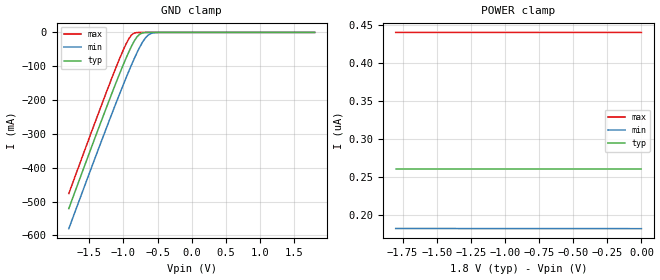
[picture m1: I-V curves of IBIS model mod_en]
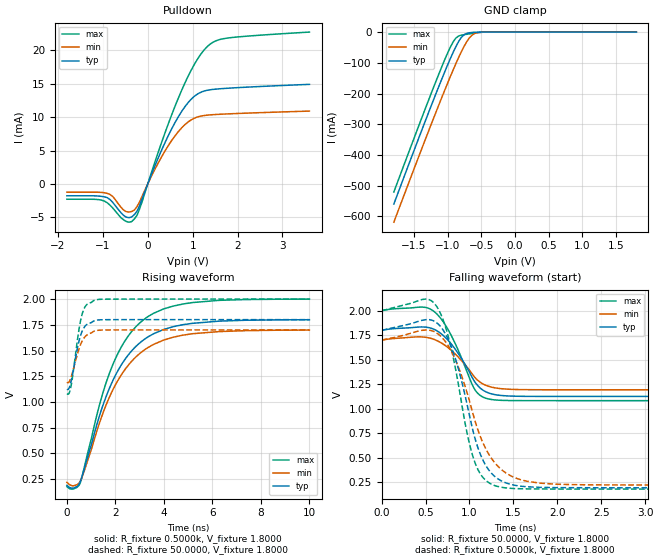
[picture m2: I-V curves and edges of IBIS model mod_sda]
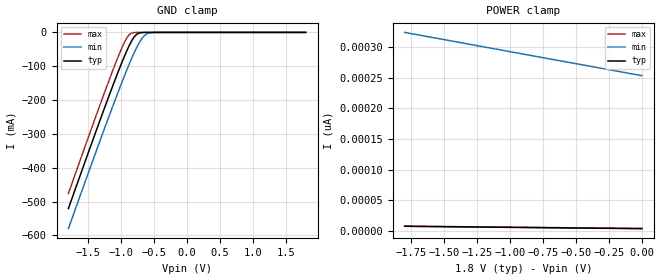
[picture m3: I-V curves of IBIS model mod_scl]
| IBIS (I/O, Buffer, Information, Specification) Model, officially
| electronic behavioral standard for Buffer structures of digital pins.
[IBIS ver]  4.0
[File name] m24c32_g4_tssop8.ibs
[File Rev]  1.0
[Date]   10 Apr 2015
[Source]   CAD & Design Services (Catania) - STMicroelectronics
[Notes]
   (Note1)  This IBIS model includes the TSSOP8 package data
   (Note2)  This IBIS model has some Notes about the non-monotonicity
   of the I-V curves, but they are not indicative of problems
   inside the model;
[Copyright] (c) 2015 STMicroelectronics
|   Component M24C32
[Component] M24C32
[Manufacturer] STMicroelectronics
[Package]
| variable   typ   min   max
R_pkg   0.0   0.0   0.0
L_pkg   0.0H   0.0H   0.0H
C_pkg   0.0F   0.0F   0.0F
[Pin]  signal_name   model_name   R_pin   L_pin   C_pin
1   E0   mod_en   NA   NA   NA
2   E1   mod_en   NA   NA   NA
3   E2   mod_en   NA   NA   NA
4   VSS   GND   NA   NA   NA
5   SDA   mod_sda   NA   NA   NA
6   SCL   mod_scl   NA   NA   NA
7   WCN   mod_wcn   NA   NA   NA
8   VCC   POWER   NA   NA   NA
[Package Model]  182696_TSSOP8
[Define Package Model]  182696_TSSOP8
[Manufacturer]  STMicroelectronics
[OEM]  STMicroelectronics
[Description]  8 pin TSSOP package
[Number Of Pins]  8
[Pin Numbers]
|Pin Num   Terminal Name
1   | net1
2   | net2
3   | net3
4   | net4_GND
5   | net5
6   | net6
7   | net7
8   | net8_VDD
[Model Data]
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[End Model Data]
[End Package Model]
| Models and submodels in the file (4): mod_en (Input), mod_sda (I/O_open_drain), mod_scl (Input), mod_wcn (Input)
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|   Model mod_en
[Model]   mod_en
Model_type Input
Vinl   =   0.540V
Vinh   =   1.260V
C_comp   2.193pF   2.023pF   2.323pF
[Temperature Range]  25.0000   0.1050k   -40.0000
[Voltage Range]   1.8000V   1.7000V   2.0000V
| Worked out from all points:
|   GND clamp passes 1 mA (typ) near -0.70 V on its own axis
[GND_clamp]
|Voltage   I(typ)   I(min)   I(max)
-1.8V     -520.9mA   -580.3mA   -476.4mA
-1.2V     -196.3mA   -256.7mA   -150.7mA
-1.04V    -114.2mA   -173.9mA   -69.64mA
-960mV    -75.48mA   -133.8mA   -33.45mA
-880mV    -40.17mA   -95.3mA    -7.265mA
-800mV    -12.91mA   -59.47mA   -440.5uA
-760mV    -5.098mA   -43.24mA   -160.1uA
-720mV    -1.558mA   -28.78mA   -103.5uA
-640mV    -123uA     -8.384mA   -71.39uA
-560mV    -21.07uA   -1.285mA   -48.43uA
-480mV    -9.394uA   -158.8uA   -27.66uA
1.8V      261.1nA    182.5nA    398.6nA
[POWER_clamp]
|Voltage   I(typ)   I(min)   I(max)
-1.8V     261.1nA    182.6nA    440.6nA
-1.36V    261.1nA    182.6nA    440.6nA
-1.34V    261.1nA    182.5nA    440.6nA
-620mV    261.1nA    182.5nA    440.6nA
-600mV    261.1nA    182.5nA    440.5nA
-100mV    261.1nA    182.5nA    440.5nA
-80mV     261.1nA    182.4nA    440.5nA
0V        261.1nA    182.4nA    440.5nA
|   Model mod_sda
[Model]   mod_sda
Model_type I/O_open_drain
Polarity   Non-Inverting
Vinl  =   0.540V
Vinh  =   1.260V
Vmeas  =   0.900V
Cref   =   10pF
Rref   =   1k
Vref   =   1.800V
C_comp   2.925pF   2.793pF   3.207pF
[Temperature Range]  25.0000   0.1050k   -40.0000
[Voltage Range]   1.8000V   1.7000V   2.0000V
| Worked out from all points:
|   slope of the pulldown table from 0 to 0.27 V, typ, clamps not added: 60.4 ohm
|   GND clamp passes 1 mA (typ) near -0.63 V on its own axis
|   rising waveform, R_fixture 0.5000k, V_fixture 1.8000: 20-80 % time 1.69ns typ, 1.72ns min, 1.62ns max; typ from 0.191 V to 1.8 V
|   rising waveform, R_fixture 50.0000, V_fixture 1.8000: 20-80 % time 367ps typ, 406ps min, 342ps max; typ from 1.12 V to 1.8 V
|   falling waveform, R_fixture 50.0000, V_fixture 1.8000: 20-80 % time 285ps typ, 301ps min, 272ps max; typ from 1.8 V to 1.12 V
|   falling waveform, R_fixture 0.5000k, V_fixture 1.8000: 20-80 % time 284ps typ, 351ps min, 243ps max; typ from 1.8 V to 0.191 V
[Pulldown]
|Voltage   I(typ)   I(min)   I(max)
-1.8V     -1.768mA   -1.24mA    -2.288mA
-900mV    -2.056mA   -1.416mA   -2.828mA
-780mV    -2.755mA   -1.875mA   -3.588mA
-540mV    -4.691mA   -3.894mA   -5.355mA
-360mV    -4.947mA   -4.125mA   -5.641mA
-180mV    -3.208mA   -2.663mA   -3.707mA
240mV     4mA        3.219mA    4.882mA
660mV     9.81mA     7.657mA    12.5mA
1.02V     13.01mA    9.782mA    17.68mA
1.32V     14.01mA    10.29mA    20.52mA
1.74V     14.3mA     10.47mA    21.79mA
3.6V      14.9mA     10.9mA     22.72mA
[GND_clamp]
|Voltage   I(typ)   I(min)   I(max)
-1.8V     -560mA     -619.1mA   -520.9mA
-1.24V    -237mA     -297.3mA   -196.5mA
-1.08V    -148.5mA   -208.5mA   -108.4mA
-960mV    -85.65mA   -144.1mA   -48.54mA
-880mV    -47.76mA   -103.1mA   -19.64mA
-800mV    -18.02mA   -64.94mA   -10.12mA
-760mV    -9.035mA   -47.59mA   -8.516mA
-720mV    -4.395mA   -32.1mA    -7.15mA
-640mV    -1.177mA   -9.975mA   -4.574mA
-560mV    -260.9uA   -1.867mA   -2.212mA
-440mV    -32.49uA   -185.8uA   -105.6uA
1.8V      82.25pA    1.254nA    77.12pA
[Ramp]
| variable   typ   min   max
dV/dt_r  0.4056/0.4701n   0.3050/0.5615n   0.5515/0.4211n
dV/dt_f  0.4056/0.3622n   0.3050/0.3797n   0.5515/0.3052n
R_load = 50.0000
[Rising Waveform]
R_fixture= 0.5000k
V_fixture= 1.8000
V_fixture_min= 1.7000
V_fixture_max= 2.0000
|time   V(typ)   V(min)   V(max)
0s        191mV      219.5mV    177.6mV
270ps     163.8mV    185.7mV    155.2mV
540ps     218.9mV    224.9mV    208mV
1.34ns    863.1mV    794.3mV    968.7mV
1.8ns     1.159V     1.072V     1.308V
2.46ns    1.436V     1.336V     1.618V
3.16ns    1.603V     1.5V       1.799V
3.98ns    1.704V     1.601V     1.904V
5.18ns    1.764V     1.663V     1.966V
10ns      1.799V     1.699V     1.999V
[Rising Waveform]
R_fixture= 50.0000
V_fixture= 1.8000
V_fixture_min= 1.7000
V_fixture_max= 2.0000
|time   V(typ)   V(min)   V(max)
0s        1.124V     1.192V     1.081V
100ps     1.14V      1.199V     1.09V
180ps     1.21V      1.247V     1.166V
260ps     1.305V     1.313V     1.289V
480ps     1.571V     1.502V     1.677V
560ps     1.643V     1.556V     1.786V
640ps     1.694V     1.597V     1.863V
800ps     1.749V     1.646V     1.941V
1.14ns    1.79V      1.689V     1.988V
10ns      1.8V       1.7V       2V
[Falling Waveform]
R_fixture= 50.0000
V_fixture= 1.8000
V_fixture_min= 1.7000
V_fixture_max= 2.0000
|time   V(typ)   V(min)   V(max)
0s        1.8V       1.7V       2V
450ps     1.833V     1.732V     2.036V
590ps     1.811V     1.708V     1.995V
690ps     1.755V     1.664V     1.9V
790ps     1.662V     1.597V     1.75V
910ps     1.51V      1.489V     1.515V
1.07ns    1.261V     1.31V      1.182V
1.15ns    1.19V      1.253V     1.119V
1.29ns    1.143V     1.212V     1.088V
10ns      1.124V     1.192V     1.081V
[Falling Waveform]
R_fixture= 0.5000k
V_fixture= 1.8000
V_fixture_min= 1.7000
V_fixture_max= 2.0000
|time   V(typ)   V(min)   V(max)
0s        1.8V       1.7V       2V
620ps     1.88V      1.775V     2.051V
720ps     1.772V     1.69V      1.853V
820ps     1.562V     1.537V     1.5V
960ps     1.094V     1.199V     803.6mV
1.06ns    705.6mV    883.4mV    454.4mV
1.18ns    428.5mV    599.9mV    271.9mV
1.34ns    273.9mV    397mV      201.4mV
2.16ns    192.5mV    224mV      178.4mV
10ns      191mV      219.5mV    177.6mV
|   Model mod_scl
[Model]   mod_scl
Model_type Input
Vinl   =   0.540V
Vinh   =   1.260V
C_comp   2.193pF   2.023pF   2.323pF
[Temperature Range]  25.0000   0.1050k   -40.0000
[Voltage Range]   1.8000V   1.7000V   2.0000V
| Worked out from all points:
|   GND clamp passes 1 mA (typ) near -0.70 V on its own axis
[GND_clamp]
|Voltage   I(typ)   I(min)   I(max)
-1.8V     -520.5mA   -579.9mA   -476.1mA
-1.24V    -217.2mA   -277.5mA   -171.5mA
-1.08V    -134.2mA   -194.1mA   -89.03mA
-960mV    -75.37mA   -133.6mA   -33.28mA
-880mV    -40.08mA   -95.18mA   -7.121mA
-800mV    -12.85mA   -59.37mA   -321.2uA
-760mV    -5.046mA   -43.15mA   -53.02uA
-720mV    -1.515mA   -28.7mA    -8.596uA
-640mV    -95.71uA   -8.329mA   -224.5nA
-560mV    -5.562uA   -1.25mA    -5.861nA
-480mV    -321.5nA   -139.5uA   -153.9pA
1.8V      3.691pA    257.4pA    3.633pA
[POWER_clamp]
|Voltage   I(typ)   I(min)   I(max)
-1.8V     7.58pA     324.2pA    7.783pA
-700mV    5.176pA    280.9pA    5.483pA
-680mV    5.133pA    280.2pA    5.442pA
0V        3.691pA    253.5pA    4.042pA
